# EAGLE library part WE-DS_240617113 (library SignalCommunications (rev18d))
WE-DS D-SUB-Filter Connectors Bent 90° Characteristics Standard type filtered with 1000 pF High attenuation of more than 40 dB @ 180 MHz Low size: 6.3 mm Rated voltage: 125 VDC Rated current @ 20 ºC: 5 A Withstand voltage: 250 VRMS Insulation resistance: min. 1000 MΩ Operating temperature: –55 ºC to +125 ºC Applications Filtering of interfaces External connection to -printer -sensor -display Details see: http://katalog.we-online.de/en/pbs/D-SUB-Filter Bent 90° Created on 2015-05-04 2015 (C) Wurth Elektronik
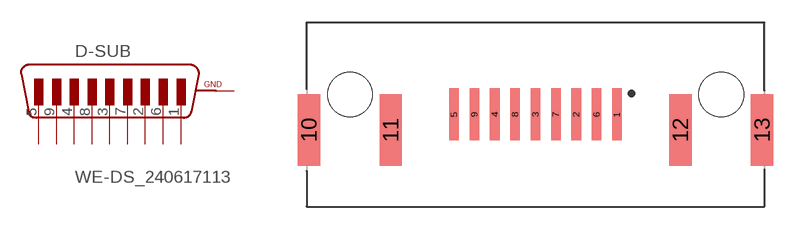
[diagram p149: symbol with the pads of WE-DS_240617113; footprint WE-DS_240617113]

Designator prefix D-SUB

## WE-DS_240617113 (WE-NUMBER: 240617113/9pins_female)  [WE-DS_240617113]
1  5  pas
2  4  pas
3  3  pas
4  2  pas
5  1  pas
6  9  pas
7  8  pas
8  7  pas
9  6  pas
10  GND  pwr
11  GND  pwr
12  GND  pwr
13  GND  pwr

## Footprint WE-DS_240617113 (pad centres in mm)
smd 0.65 x 3.5: 1 5.48,0; 2 2.74,0; 3 0,0; 4 -2.74,0; 5 -5.48,0; 6 4.11,0; 7 1.37,0; 8 -1.37,0; 9 -4.11,0
smd 1.5 x 4.8: 10 -15.25,-1.05; 11 -9.75,-1.05; 12 9.75,-1.05; 13 15.25,-1.05
hole 3 at -12.5,1.35
hole 3 at 12.5,1.35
